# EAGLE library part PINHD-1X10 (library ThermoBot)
PIN HEADER
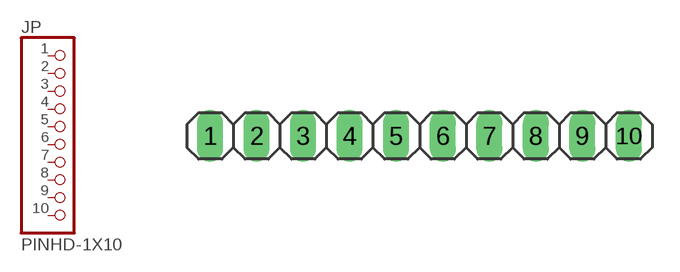
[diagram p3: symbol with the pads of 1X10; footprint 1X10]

Designator prefix JP

## PINHD-1X10TH  [1X10]
1  1  pas
2  2  pas
3  3  pas
4  4  pas
5  5  pas
6  6  pas
7  7  pas
8  8  pas
9  9  pas
10  10  pas

## Footprint 1X10 (pad centres in mm)
PIN HEADER
drill 0.85 pad 1.422 long: 1 -11.43,0; 2 -8.89,0; 3 -6.35,0; 4 -3.81,0; 5 -1.27,0; 6 1.27,0; 7 3.81,0; 8 6.35,0; 9 8.89,0; 10 11.43,0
